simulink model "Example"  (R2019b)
settings: Solver=VariableStepAuto  StartTime=0.0  StopTime=inf  RelTol=1e-3
libraries: dspsrcs4 x3

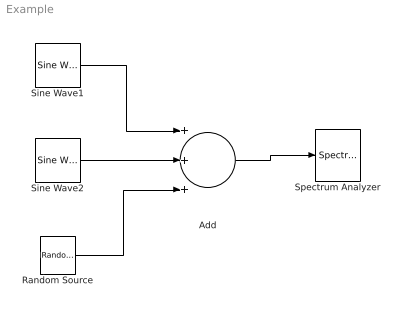
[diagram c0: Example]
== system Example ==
  Add : Sum  Inputs=+++
  Random Source : dspsrcs4/Random Source  SrcType=Gaussian  NormMethod=Ziggurat  CltLength=12  MinVal=0  MaxVal=1  MeanVal=0  VarVal=0.05  RepMode=Not repeatable  rawSeed=1  IsInherit=off  SampMode=Discrete  SampTime=1  SampFrame=1  DataType=Double  OutComplex=Real  OutputFrames=off
  Sine Wave1 : dspsrcs4/Sine Wave  Amplitude=1  Frequency=1e3  Phase=0  SampleMode=Discrete  OutComplex=Complex  CompMethod=Trigonometric fcn  TableSize=Speed  SampleTime=1/1000  SamplesPerFrame=1  ResetState=Restart at time zero  OutputFrames=off  dataType=double  wordLen=16  udDataType=sfix(16)  fracBitsMode=Best precision  numFracBits=15  OutDataTypeStr=double  LastOutDataTypeStr=double
  Sine Wave2 : dspsrcs4/Sine Wave  Amplitude=1  Frequency=15e3  Phase=0  SampleMode=Discrete  OutComplex=Complex  CompMethod=Trigonometric fcn  TableSize=Speed  SampleTime=1/1000  SamplesPerFrame=1  ResetState=Restart at time zero  OutputFrames=off  dataType=double  wordLen=16  udDataType=sfix(16)  fracBitsMode=Best precision  numFracBits=15  OutDataTypeStr=double  LastOutDataTypeStr=double
  Spectrum Analyzer : SpectrumAnalyzer
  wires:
  Sine Wave1/1 -> Add/1
  Sine Wave2/1 -> Add/2
  Random Source/1 -> Add/3
  Add/1 -> Spectrum Analyzer/1
